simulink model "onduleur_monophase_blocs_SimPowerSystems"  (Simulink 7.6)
settings: Solver=FixedStepDiscrete  StartTime=0.0  StopTime=0.025  RelTol=1e-3
InitFcn:
  | clc
  | clear all
  | close all
  | Ts=5e-5;
undefined symbols (not defined in the file or in its folder): arm, bridge, pulses
libraries: powerlib x10, powerlib_extras x2

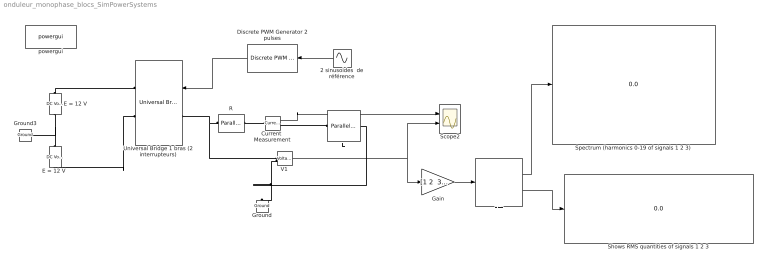
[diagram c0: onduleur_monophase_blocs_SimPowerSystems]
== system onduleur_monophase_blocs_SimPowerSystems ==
  2 sinusoides  de référence : Sin  Frequency=2*pi*60  SampleTime=Ts
  Current  Measurement : powerlib/Measurements/Current Measurement  DialogController=POWERSYS.PowerSysDialog  SystemSampleTime=-1  PhasorSimulation=off  OutputType=Complex  PSBequivalent=0
  Discrete PWM Generator 2 pulses : powerlib_extras/Discrete  Control Blocks/Discrete PWM Generator  DialogController=POWERSYS.PowerSysDialog  SystemSampleTime=-1  GeneratorMode="1-arm  bridge (2 pulses)"  Fc=1080  Ts=5e-5  Internal=off  mIndex=0.8  Freq=60  Phase=0
  E = 12 V : powerlib/Electrical Sources/DC Voltage Source  Description=source block  DialogController=POWERSYS.PowerSysDialog  SystemSampleTime=-1  Amplitude=12  Measurements=None
  "E = 12 V " : powerlib/Electrical Sources/DC Voltage Source  Description=source block  DialogController=POWERSYS.PowerSysDialog  SystemSampleTime=-1  Amplitude=12  Measurements=None
  FFT : powerlib_extras/Discrete Measurements/FFT  DialogController=POWERSYS.PowerSysDialog  SystemSampleTime=-1  Nsig=3  f1=60  Ts=Ts  TsFFT=0.1  base="[1 1  1   ]"  nDec=0  SPSmask="[1 -1  1  ]"  figure_N=2
  Gain : Gain  Gain="[1 2  3 ]"
  Ground : powerlib/Elements/Ground  DialogController=POWERSYS.PowerSysDialog  PhysicalDomain=powersysdomain  SubClassName=unknown  LeftPortType=p1  RightPortType=p1  LConnTagsString=a
  Ground3 : powerlib/Elements/Ground  DialogController=POWERSYS.PowerSysDialog  PhysicalDomain=powersysdomain  SubClassName=unknown  LeftPortType=p1  RightPortType=p1  LConnTagsString=a
  L : powerlib/Elements/Parallel RLC Branch  DialogController=POWERSYS.PowerSysDialog  PhysicalDomain=powersysdomain  SubClassName=unknown  LeftPortType=p1  RightPortType=p1  LConnTagsString=a  RConnTagsString=__new0  BranchType=L  Resistance=1  Inductance=0.1  SetiL0=off  InitialCurrent=0  Capacitance=1e-6  Setx0=off  InitialVoltage=0  Measurements=None
  R : powerlib/Elements/Parallel RLC Branch  DialogController=POWERSYS.PowerSysDialog  PhysicalDomain=powersysdomain  SubClassName=unknown  LeftPortType=p1  RightPortType=p1  LConnTagsString=a  RConnTagsString=__new0  BranchType=R  Resistance=10  Inductance=1.0  SetiL0=off  InitialCurrent=0  Capacitance=25e-06  Setx0=off  InitialVoltage=0  Measurements=Branch voltage and current
  Scope2 : Scope  NumInputPorts=2
  Shows RMS quantities of signals 1 2 3 : Display
  Spectrum (harmonics 0-19 of signals 1 2 3) : Display
  Universal Bridge 1 bras (2 interrupteurs) : powerlib/Power Electronics/Universal Bridge  DialogController=POWERSYS.PowerSysDialog  SystemSampleTime=-1  Arms=1  SnubberResistance=10000  SnubberCapacitance=inf  Device=MOSFET / Diodes  Ron=1e-4  Lon=0  ForwardVoltages="[  1  1  ]"  ForwardVoltage=.8  GTOparameters=[ 10e-6 , 20e-6 ]  IGBTparameters=[ 1e-6 , 2e-6 ]  Measurements=None  Measurements_2=None  converterType=Rectifier
  V1 : powerlib/Measurements/Voltage Measurement  Tag=PoWeRsYsTeMmEaSuReMeNt  DialogController=POWERSYS.PowerSysDialog  SystemSampleTime=-1  PhasorSimulation=off  OutputType=Magnitude  PSBequivalent=0
  powergui : powerlib/powergui  SystemSampleTime=-1  SimulationMode=Discrete  SampleTime=Ts  frequency=60  SPID=off  DisableSnubberDevices=off  DisableRonSwitches=off  DisableVfSwitches=off  SwTol=0  Interpol=off  frequencyindice=0  echomessages=off  HookPort=off  DisplayEquations=off  FunctionMessages=off  EnableUseOfTLC=off  x0status=blocks  RestoreLinks=warning  ResistiveCurrentMeasurement=off  Frange=[0:2:500]  Ylog=off  Xlog=on  ShowGrid=off  save=off  variable=ZData  ZoomFFT=on  StartTime=0.0  cycles=1  DisplayStyle=1  fundamental=60  FreqAxis=off  MaxFrequency=1000  frequencyindicesteady=1  RmsSteady=1  display=off  Ts=0  methode=off
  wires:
  Discrete PWM Generator 2 pulses/1 -> Universal Bridge 1 bras (2 interrupteurs)/1
  2 sinusoides  de référence/1 -> Discrete PWM Generator 2 pulses/1
  Current  Measurement/1 -> Scope2/1
  V1/1 -> Scope2/2, Gain/1
  FFT/2 -> Shows RMS quantities of signals 1 2 3/1
  FFT/1 -> Spectrum (harmonics 0-19 of signals 1 2 3)/1
  Gain/1 -> FFT/1
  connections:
  E = 12 V/LConn1 -- "E = 12 V "/RConn1 -- Ground3/LConn1
  Universal Bridge 1 bras (2 interrupteurs)/RConn2 -- "E = 12 V "/LConn1
  E = 12 V/RConn1 -- Universal Bridge 1 bras (2 interrupteurs)/RConn1
  R/RConn1 -- Universal Bridge 1 bras (2 interrupteurs)/LConn1 -- V1/LConn1
  R/LConn1 -- Current  Measurement/LConn1
  L/LConn1 -- Current  Measurement/RConn1
  V1/LConn2 -- Ground/LConn1 -- L/RConn1
